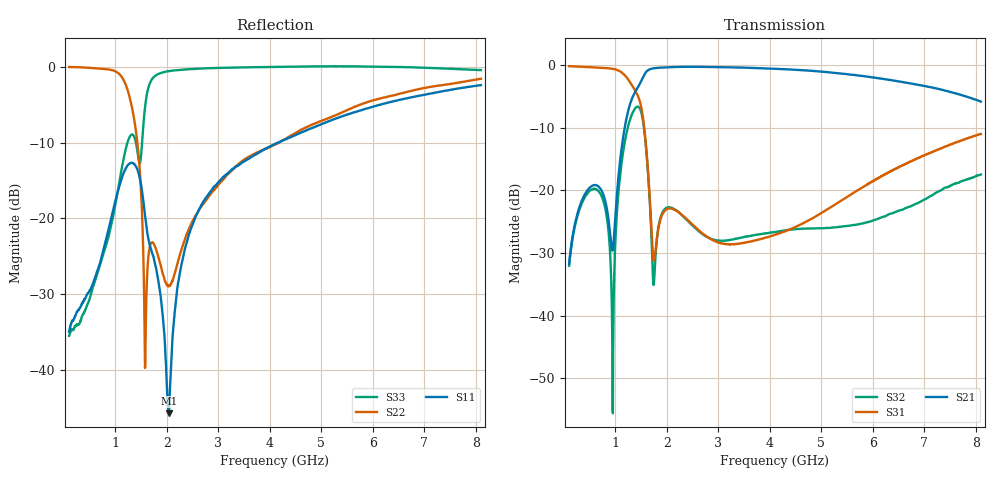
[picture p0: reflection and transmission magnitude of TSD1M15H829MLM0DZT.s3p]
# MHZ S RI R 50
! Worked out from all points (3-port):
!   1601 points, 100 MHz to 8.1 GHz, reference 50 ohm
!   strongest paths, dB at 100 MHz, 2.1 GHz, 4.1 GHz, 6.1 GHz, 8.1 GHz:
!     S21: -31.7, -0.3, -0.6, -2.1, -5.8
!     S31: -0.2, -22.9, -27.1, -18.0, -11.0
!     S32: -32.0, -22.8, -26.6, -24.5, -17.5
!   lowest |S11| = -45.7 dB at 2.035 GHz (marker M1), VSWR 1.01, Z = 50.4 + j0.36 ohm
!   |S11| at or under -10 dB: start of sweep to 4.149 GHz
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100  0.0177 0.00239  0.00224 0.0258  0.97 -0.145
     0.00224 0.0259  0.986 -0.169  0.00579 0.0246
     0.971 -0.145  0.00583 0.0244  0.0167 0.00186
670  0.0424 -0.0207  0.0594 0.0894  0.494 -0.818
     0.0593 0.0899  0.327 -0.921  0.0987 -0.0054
     0.494 -0.818  0.0986 -0.00501  0.0449 0.00854
950  0.0728 -0.0849  -0.0166 0.0296  -0.0217 -0.934
     -0.0165 0.0297  -0.354 -0.883  -0.000644 0.00147
     -0.0218 -0.935  -0.000787 0.00147  0.1 0.0166
1350  -0.19 -0.132  -0.341 0.466  -0.629 -0.206
      -0.341 0.464  -0.403 0.263  0.432 -0.0141
      -0.628 -0.206  0.43 -0.0157  0.0837 -0.344
1565  -0.0999 0.0503  -0.162 0.831  -0.193 0.231
      -0.163 0.83  0.0169 0.00945  -0.0906 -0.274
      -0.193 0.231  -0.0933 -0.275  0.303 0.404
1745  -0.0488 0.0243  0.197 0.925  -0.0267 0.00658
      0.197 0.924  -0.0609 -0.0301  0.00415 -0.0171
      -0.0267 0.00655  0.00412 -0.0173  0.742 -0.433
2035  0.00374 0.00357  0.521 0.81  -0.0616 -0.037
      0.521 0.81  -0.0143 -0.0333  0.0501 -0.0534
      -0.0616 -0.0369  0.0506 -0.0535  0.223 -0.912
2550  0.0489 -0.0889  0.787 0.566  -0.0509 0.00352
      0.787 0.567  0.0607 -0.084  0.024 -0.0444
      -0.051 0.00351  0.0238 -0.0441  -0.338 -0.913
4100  -0.0352 -0.309  0.937 0.0221  -0.0123 0.0426
      0.935 0.0247  0.0373 -0.306  0.0245 -0.0402
      -0.0122 0.0426  0.024 -0.04  -0.887 -0.465
8100  -0.744 -0.152  0.27 -0.432  -0.0195 0.281
      0.265 -0.438  -0.634 -0.545  -0.101 0.093
      -0.0197 0.282  -0.0987 0.0908  -0.922 0.248
